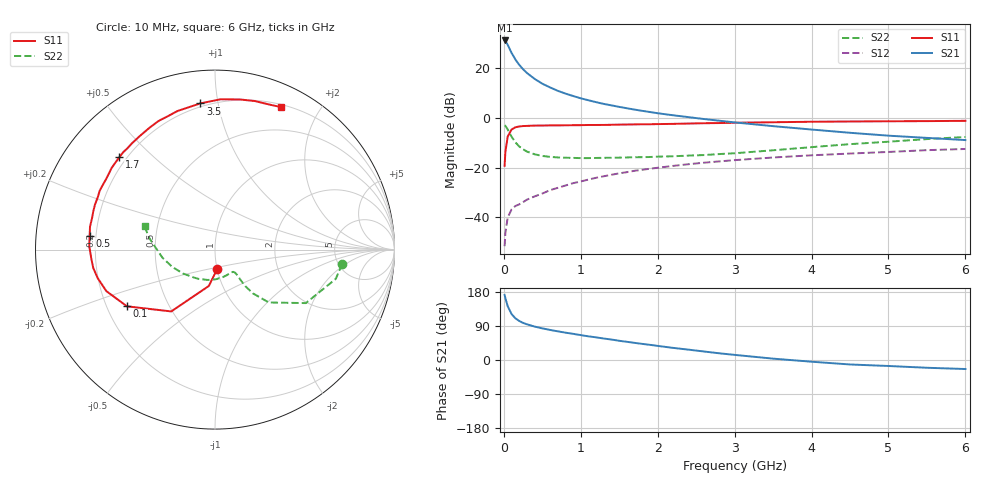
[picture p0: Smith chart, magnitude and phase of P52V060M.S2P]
! SIEMENS Small Signal Semiconductors
! BFP183
! Si NPN RF Bipolar Junction Transistor in SOT143
! VCE = 2 V  IC = 60 mA
! Common Emitter S-Parameters:  March  1996
# GHz  S  MA  R  50
!  f  S11  S21  S12  S22
! GHz  MAG  ANG  MAG  ANG  MAG  ANG  MAG  ANG
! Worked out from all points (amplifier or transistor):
!   36 points, 10 MHz to 6 GHz, reference 50 ohm
!   highest |S21| = 31.2 dB at 10 MHz (marker M1)
!   |S21| within 3 dB of that: start of sweep to 69.45 MHz
!   unconditionally stable (mu >= 1): start of sweep to 36.47 MHz; 165.3 MHz to end of sweep
!   at 250 MHz: K = 1.24, MAG = 23.9 dB, |S12| = -33.9 dB
!   at 1.4 GHz: K = 1.76, MAG = 8.9 dB, |S12| = -22.9 dB
!   at 6 GHz: K = 1.39, MAG = -1.9 dB, |S12| = -12.5 dB
!   S11 on the Smith chart (normalised r, x): 10 MHz: 1.00, -0.22; 100 MHz: 0.28, -0.27; 500 MHz: 0.18, +0.05; 1.7 GHz: 0.17, +0.39; 3.5 GHz: 0.18, +0.89; 6 GHz: 0.23, +1.54
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0.01  0.1086 -83.4  36.47 171.5  0.0026 60.0  0.7132 -6.5
0.02  0.2059 -99.7  35.48 163.3  0.0048 66.9  0.6925 -13.6
0.05  0.4221 -125.3  29.87 142.0  0.0098 60.2  0.5873 -30.5
0.1  0.5835 -147.2  20.54 121.3  0.0143 48.3  0.4204 -44.5
0.15  0.6481 -159.1  15.09 110.0  0.0168 45.4  0.3224 -49.1
0.2  0.6725 -166.3  11.75 103.0  0.0181 46.0  0.2664 -50.3
0.25  0.686 -171.4  9.584 97.9  0.0201 48.3  0.2335 -50.1
0.3  0.6908 -175.7  8.069 94.2  0.0225 50.7  0.2102 -49.6
0.4  0.7009 178.4  6.122 88.2  0.0262 54.8  0.185 -48.9
0.5  0.7026 173.8  4.899 83.5  0.0299 56.4  0.1713 -49.0
0.6  0.708 169.6  4.13 79.4  0.035 59.3  0.1643 -49.7
0.7  0.7071 165.8  3.524 75.7  0.0389 60.6  0.1599 -50.9
0.9  0.7142 159.5  2.768 69.1  0.0484 61.3  0.1565 -55.1
1.1  0.7213 153.0  2.27 62.4  0.0573 61.6  0.1551 -60.0
1.3  0.7228 147.1  1.915 56.6  0.0668 60.3  0.1572 -65.8
1.7  0.741 135.9  1.473 45.2  0.0861 57.9  0.1614 -78.7
2.2  0.7593 123.3  1.132 32.0  0.108 52.9  0.1686 -96.6
2.8  0.7886 109.3  0.879 17.7  0.133 46.4  0.1869 -118.9
3.5  0.8186 95.7  0.683 3.6  0.1594 39.1  0.223 -143.4
4.5  0.8479 80.6  0.502 -11.8  0.1916 28.4  0.2963 -171.3
5.5  0.8628 69.6  0.396 -20.5  0.2241 18.7  0.3747 169.5
6  0.8746 65.2  0.358 -23.8  0.2368 13.5  0.4133 161.6
